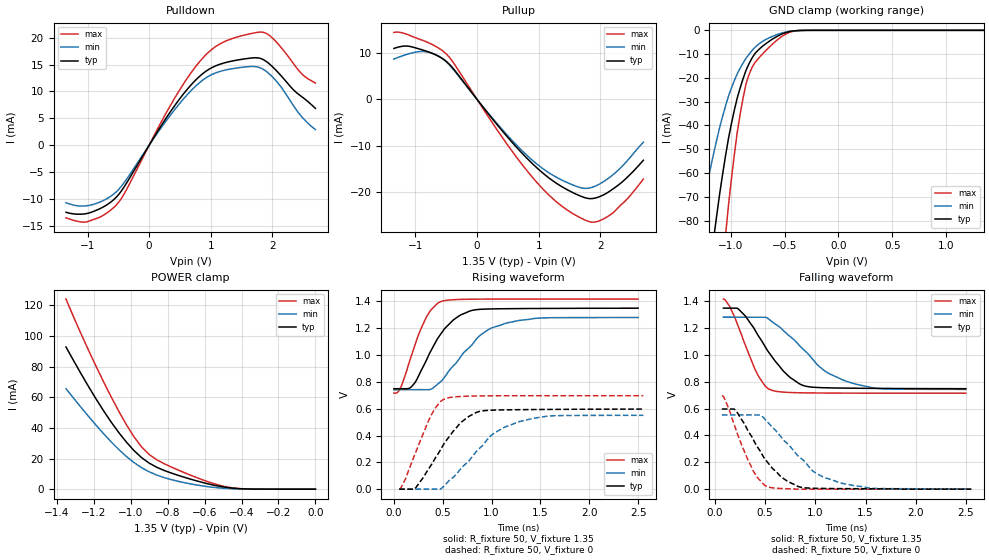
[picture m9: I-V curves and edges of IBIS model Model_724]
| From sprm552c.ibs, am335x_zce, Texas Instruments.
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| Model based on original model for BCSHTLTCSCDDVPBFZ_SSDHV
|   Sub model SR11_6MA_PADP_5PER_1P35
[model]   Model_724
|[Description]  [1.35V-3-STATE-NOTERM-SR11:6MA, IND, 5%]
|   Slowest slew rate (SR[1:0] = "11"), 1.33 * RExt = 0.750 * Iout
|   (I[2:0] = "001"), 6mA nominal with Rext = 50R,ODT off (ODT[1:0]
|   = "00") CMOS mode,Industrial temperature range (-40C to 125C,
|   25C nominal),5% power supply tolerance
|[Input Load]   NOTERM
|[Output Drive] SR11:6MA
|Voltage   1.35V
|Mode   3-STATE
Model_type   3-state
Polarity   Non-Inverting
Enable   Active-Low
Cref =  15pF
Rref =  100.0000M
Vref =  0V
Vmeas =  0.675
C_comp   1.865048p   1.679967p   1.989968p
[Temperature Range]   25   125   -40
[Voltage Range]   1.35   1.2825   1.4175
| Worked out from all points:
|   slope of the pulldown table from 0 to 0.203 V, typ, clamps not added: 53.9 ohm
|   slope of the pullup table from 0 to 0.203 V, typ, clamps not added: 58.7 ohm
|   GND clamp passes 1 mA (typ) near -0.49 V on its own axis
|   POWER clamp passes 1 mA (typ) near -0.47 V on its own axis
|   rising waveform, R_fixture 50, V_fixture 1.35: 20-80 % time 297ps typ, 400ps min, 209ps max; typ from 0.749 V to 1.35 V
|   rising waveform, R_fixture 50, V_fixture 0: 20-80 % time 334ps typ, 442ps min, 236ps max; typ from 0 V to 0.597 V
|   falling waveform, R_fixture 50, V_fixture 1.35: 20-80 % time 337ps typ, 472ps min, 225ps max; typ from 1.35 V to 0.748 V
|   falling waveform, R_fixture 50, V_fixture 0: 20-80 % time 325ps typ, 425ps min, 222ps max; typ from 0.597 V to 0 V
[POWER_clamp]
-1.35V    92.75mA    65.58mA    124.1mA
-1.227V   66.81mA    47.37mA    90.43mA
-1.145V   50.92mA    36.04mA    69.8mA
-1.064V   36.83mA    25.8mA     50.7mA
-981.8mV  25.17mA    17.34mA    34.14mA
-940.9mV  20.58mA    14.01mA    27.56mA
-900mV    17mA       11.33mA    22.64mA
-859.1mV  14.3mA     9.214mA    19.2mA
-736.4mV  8.769mA    4.942mA    12.14mA
-490.9mV  1.299mA    528.4uA    1.73mA
-368.2mV  117.2uA    50.88uA    117.5uA
0V        1.028nA    11.95nA    1.029nA
[Pulldown]
-1.35V    -12.46mA   -10.69mA   -13.5mA
-1.023V   -12.73mA   -11.27mA   -14.28mA
-531.8mV  -9.642mA   -8.642mA   -11.1mA
-409.1mV  -7.802mA   -7.007mA   -9.123mA
531.8mV   9.169mA    8.275mA    10.95mA
859.1mV   13.21mA    12.02mA    16.07mA
1.145V    15.05mA    13.71mA    18.82mA
1.677V    16.25mA    14.66mA    20.83mA
1.882V    15.74mA    13.9mA     20.91mA
2.086V    13.63mA    11.64mA    18.93mA
2.495V    8.875mA    5.068mA    13.09mA
2.7V      6.853mA    2.908mA    11.56mA
[Pullup]
-1.35V    11.03mA    8.75mA     14.52mA
-1.145V   11.56mA    9.727mA    14.13mA
-900mV    10.77mA    10.38mA    12.87mA
-572.7mV  8.933mA    8.936mA    10.65mA
-409.1mV  7.026mA    6.847mA    8.416mA
736.4mV   -11.73mA   -11.18mA   -14.19mA
1.145V    -16.79mA   -15.71mA   -20.44mA
1.555V    -20.18mA   -18.53mA   -24.72mA
1.841V    -21.49mA   -19.14mA   -26.53mA
2.045V    -20.73mA   -17.88mA   -25.93mA
2.414V    -17.18mA   -13.67mA   -21.89mA
2.7V      -13.18mA   -9.274mA   -17.26mA
[GND_clamp]
-1.35V    -159.1mA   -94.77mA   -266.2mA
-1.295V   -137.7mA   -81.77mA   -230.9mA
-1.159V   -87.19mA   -51.56mA   -145.9mA
-1.132V   -77.89mA   -46.14mA   -129.9mA
-1.05V    -52.83mA   -31.84mA   -86.44mA
-1.023V   -45.55mA   -27.75mA   -73.68mA
-940.9mV  -28.44mA   -18.28mA   -42.92mA
-859.1mV  -16.79mA   -11.75mA   -22.47mA
-804.5mV  -11.72mA   -8.559mA   -15.69mA
-722.7mV  -7.324mA   -5.162mA   -10.76mA
-395.5mV  -159.1uA   -161.1uA   -232.3uA
1.35V     1.028nA    30.09nA    754.3pA
[Ramp]
dV/dt_f 0.36256278/0.33926073n 0.32688934/0.4811971n 0.42225613/0.22532992n
dV/dt_r 0.36034279/0.33577658n 0.33457039/0.4493504n 0.41939375/0.23608854n
R_load = 50
[Rising Waveform]
R_fixture = 50
V_fixture = 1.35
V_fixture_min = 1.2825
V_fixture_max = 1.4175
0s        748.5mV    741mV      716.1mV
70.07ps   749mV      741mV      759.1mV
202.5ps   782.3mV    741.2mV    1.048V
338.4ps   972.4mV    741.3mV    1.29V
479.6ps   1.157V     801.1mV    1.398V
612ps     1.264V     921mV      1.413V
770.8ps   1.327V     1.054V     1.416V
940.6ps   1.343V     1.177V     1.417V
1.135ns   1.346V     1.235V     1.417V
2.5ns     1.349V     1.28V      1.418V
[Rising Waveform]
R_fixture = 50
V_fixture = 0
V_fixture_min = 0
V_fixture_max = 0
54.09ps   0V         0V         0V
218.3ps   6.377mV    0V         265.5mV
383.5ps   181.3mV    0V         554.5mV
526ps     352.6mV    34.86mV    675mV
681.1ps   493.4mV    150mV      691.2mV
836.8ps   570.1mV    274.6mV    694.9mV
1.01ns    589.2mV    408.9mV    696.2mV
1.266ns   592.7mV    499.8mV    696.8mV
1.612ns   594.8mV    546.6mV    697mV
2.554ns   597.3mV    550.7mV    697mV
[Falling Waveform]
R_fixture = 50
V_fixture = 1.35
V_fixture_min = 1.2825
V_fixture_max = 1.4175
83.62ps   1.349V     1.282V     1.417V
152.9ps   1.349V     1.282V     1.352V
288.5ps   1.302V     1.282V     1.1V
432.2ps   1.142V     1.282V     843.8mV
558.5ps   995.9mV    1.254V     738.8mV
860ps     778mV      1.055V     718mV
1.082ns   755.8mV    888.2mV    716.2mV
1.3ns     752.8mV    806.3mV    715.5mV
1.644ns   750.7mV    749.2mV    715.1mV
2.5ns     748.5mV    743.5mV    715.1mV
[Falling Waveform]
R_fixture = 50
V_fixture = 0
V_fixture_min = 0
V_fixture_max = 0
68.29ps   597.3mV    553.3mV    696.1mV
132.1ps   597.3mV    553.3mV    613.1mV
207ps     587mV      553.3mV    446.2mV
379.7ps   373mV      553.3mV    138mV
521.6ps   202.5mV    501.3mV    18.96mV
825.3ps   20.7mV     250.2mV    0V
992.6ps   6.463mV    126.1mV    0V
1.234ns   4.147mV    49.75mV    0V
1.585ns   2.691mV    6.049mV    0V
2.554ns   0V         2.624mV    0V
